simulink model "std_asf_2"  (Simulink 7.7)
settings: Solver=ode45  StartTime=0.0  StopTime=10.0  RelTol=1e-3

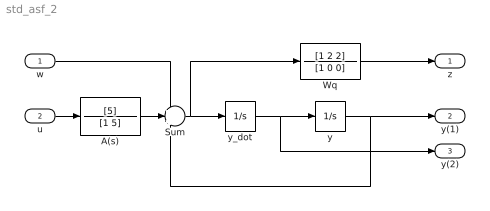
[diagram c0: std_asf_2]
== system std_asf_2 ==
  w : Inport
  u : Inport  Port=2
  A(s) : TransferFcn  Numerator=[5]  Denominator=[1 5]
  Sum : Sum  Inputs=+++
  Wq : TransferFcn  Numerator=[1 2 2]  Denominator=[1 0 0]
  y : Integrator
  y_dot : Integrator  InitialCondition=-1
  z : Outport
  y(1) : Outport  Port=2
  y(2) : Outport  Port=3
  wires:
  Sum/1 -> y_dot/1, Wq/1
  y_dot/1 -> y/1, y(2)/1
  y/1 -> y(1)/1, Sum/3
  Wq/1 -> z/1
  w/1 -> Sum/1
  u/1 -> A(s)/1
  A(s)/1 -> Sum/2
